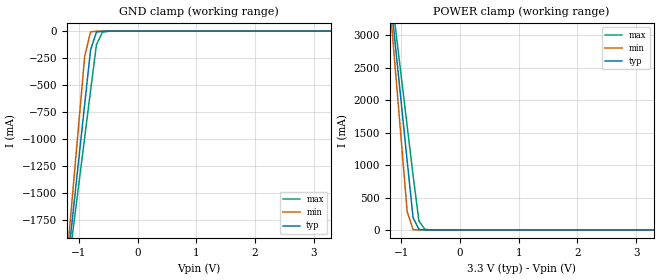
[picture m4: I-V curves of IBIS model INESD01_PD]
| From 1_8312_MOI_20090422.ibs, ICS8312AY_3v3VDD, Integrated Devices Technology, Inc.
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[Model] INESD01_PD
Model_type   Input
Polarity   Non-Inverting
Vinl = 0.80V
Vinh = 2.0V
|   typ   min   max
C_comp   2pF   1.5pF   2.5pF
|   typ   min   max
[Voltage range]  3.3V   3.15V   3.45V
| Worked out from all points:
|   GND clamp passes 1 mA (typ) near -0.55 V on its own axis
|   POWER clamp passes 1 mA (typ) near -0.60 V on its own axis
[GND_clamp]
|Voltage I(typ)   I(min)   I(max)
-3.3V     -12.83A    -15.14A    -11.37A
-1.2V     -2.195A    -2.092A    -2.281A
-1.1V     -1.689A    -1.472A    -1.849A
-900mV    -678.5mA   -232.6mA   -984.8mA
-800mV    -173.9mA   -7.175mA   -553.2mA
-700mV    -9.696mA   -1.052mA   -126mA
-600mV    -1.629mA   -178uA     -11.07mA
-300mV    -10.53uA   -5.678uA   -86.08uA
3.3V      71.13uA    62.11uA    77.58uA
[POWER_clamp]
|Voltage   I(typ)   I(min)   I(max)
-3.3V     22.38A     26.45A     19.82A
-1.2V     3.723A     3.545A     3.874A
-1.1V     2.836A     2.457A     3.116A
-1V       1.949A     1.369A     2.358A
-900mV    1.063A     281.1mA    1.601A
-800mV    191.6mA    5.074mA    844mA
-700mV    8.104mA    204.3uA    138.4mA
-600mV    678.1uA    79.74uA    10.7mA
-400mV    87.44uA    69.65uA    413.2uA
3.3V      -3.041nA   -425fA     -919.9nA
